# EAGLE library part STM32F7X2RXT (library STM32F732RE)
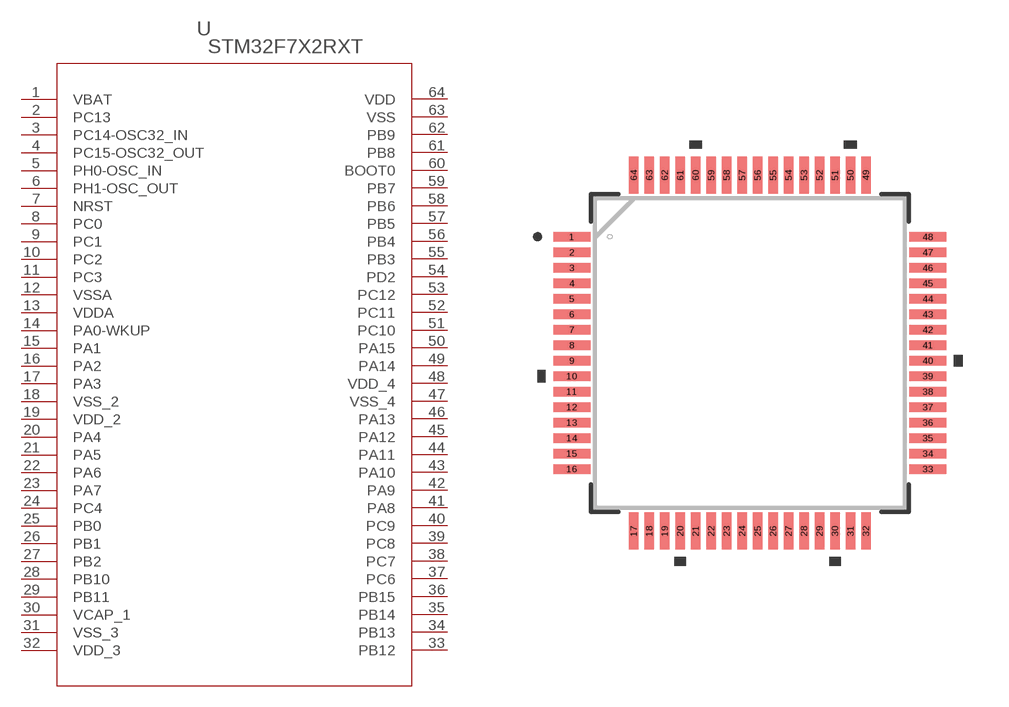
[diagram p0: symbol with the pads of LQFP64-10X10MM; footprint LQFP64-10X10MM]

Designator prefix U

## STM32F7X2RXT (MANUFACTURER_PART_NUMBER: stm32f7x2rxt; VENDOR: STMicroelectronics)  [LQFP64-10X10MM]
1  VBAT  pwr
2  PC13
3  PC14-OSC32_IN
4  PC15-OSC32_OUT
5  PH0-OSC_IN
6  PH1-OSC_OUT
7  NRST
8  PC0
9  PC1
10  PC2
11  PC3
12  VSSA  pwr
13  VDDA  pwr
14  PA0-WKUP
15  PA1
16  PA2
17  PA3
18  VSS_2  pwr
19  VDD_2  pwr
20  PA4
21  PA5
22  PA6
23  PA7
24  PC4
25  PB0
26  PB1
27  PB2
28  PB10
29  PB11
30  VCAP_1  pwr
31  VSS_3  pwr
32  VDD_3  pwr
33  PB12
34  PB13
35  PB14
36  PB15
37  PC6
38  PC7
39  PC8
40  PC9
41  PA8
42  PA9
43  PA10
44  PA11
45  PA12
46  PA13
47  VSS_4  pwr
48  VDD_4  pwr
49  PA14
50  PA15
51  PC10
52  PC11
53  PC12
54  PD2
55  PB3
56  PB4
57  PB5
58  PB6
59  PB7
60  BOOT0  in
61  PB8
62  PB9
63  VSS  pwr
64  VDD  pwr

## Footprint LQFP64-10X10MM (pad centres in mm)
smd 1.194 x 0.305: 1 -5.75,3.75; 2 -5.75,3.25; 3 -5.75,2.75; 4 -5.75,2.25; 5 -5.75,1.75; 6 -5.75,1.25; 7 -5.75,0.75; 8 -5.75,0.25; 9 -5.75,-0.25; 10 -5.75,-0.75; 11 -5.75,-1.25; 12 -5.75,-1.75; 13 -5.75,-2.25; 14 -5.75,-2.75; 15 -5.75,-3.25; 16 -5.75,-3.75; 33 5.75,-3.75; 34 5.75,-3.25; 35 5.75,-2.75; 36 5.75,-2.25; 37 5.75,-1.75; 38 5.75,-1.25; 39 5.75,-0.75; 40 5.75,-0.25; 41 5.75,0.25; 42 5.75,0.75; 43 5.75,1.25; 44 5.75,1.75; 45 5.75,2.25; 46 5.75,2.75; 47 5.75,3.25; 48 5.75,3.75
smd 0.305 x 1.194: 17 -3.75,-5.75; 18 -3.25,-5.75; 19 -2.75,-5.75; 20 -2.25,-5.75; 21 -1.75,-5.75; 22 -1.25,-5.75; 23 -0.75,-5.75; 24 -0.25,-5.75; 25 0.25,-5.75; 26 0.75,-5.75; 27 1.25,-5.75; 28 1.75,-5.75; 29 2.25,-5.75; 30 2.75,-5.75; 31 3.25,-5.75; 32 3.75,-5.75; 49 3.75,5.75; 50 3.25,5.75; 51 2.75,5.75; 52 2.25,5.75; 53 1.75,5.75; 54 1.25,5.75; 55 0.75,5.75; 56 0.25,5.75; 57 -0.25,5.75; 58 -0.75,5.75; 59 -1.25,5.75; 60 -1.75,5.75; 61 -2.25,5.75; 62 -2.75,5.75; 63 -3.25,5.75; 64 -3.75,5.75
